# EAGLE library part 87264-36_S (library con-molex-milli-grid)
RECEPTACAL
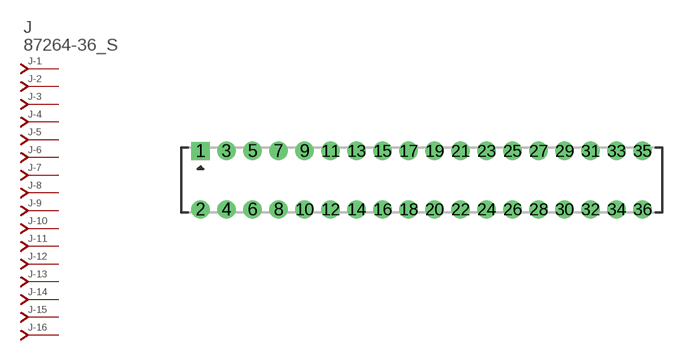
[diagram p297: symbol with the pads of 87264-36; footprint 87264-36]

Designator prefix J; gates -1=J-NV -2=J-N -3=J-N -4=J-N -5=J-N -6=J-N -7=J-N -8=J-N -9=J-N -10=J-N -11=J-N -12=J-N -13=J-N -14=J-N -15=J-N -16=J-N -17=J-N -18=J-N -19=J-N -20=J-N -21=J-N -22=J-N -23=J-N -24=J-N -25=J-N -26=J-N -27=J-N -28=J-N -29=J-N -30=J-N -31=J-N -32=J-N -33=J-N -34=J-N -35=J-N -36=J-N

## 87264-36_S  [87264-36]
1  -1:J  pas
2  -2:J  pas
3  -3:J  pas
4  -4:J  pas
5  -5:J  pas
6  -6:J  pas
7  -7:J  pas
8  -8:J  pas
9  -9:J  pas
10  -10:J  pas
11  -11:J  pas
12  -12:J  pas
13  -13:J  pas
14  -14:J  pas
15  -15:J  pas
16  -16:J  pas
17  -17:J  pas
18  -18:J  pas
19  -19:J  pas
20  -20:J  pas
21  -21:J  pas
22  -22:J  pas
23  -23:J  pas
24  -24:J  pas
25  -25:J  pas
26  -26:J  pas
27  -27:J  pas
28  -28:J  pas
29  -29:J  pas
30  -30:J  pas
31  -31:J  pas
32  -32:J  pas
33  -33:J  pas
34  -34:J  pas
35  -35:J  pas
36  -36:J  pas

## Footprint 87264-36 (pad centres in mm)
RECEPTACAL Dual Row, Side Entry
drill 0.914 square: 1 -17,2.25
drill 0.914: 2 -17,-2.25; 3 -15,2.25; 4 -15,-2.25; 5 -13,2.25; 6 -13,-2.25; 7 -11,2.25; 8 -11,-2.25; 9 -9,2.25; 10 -9,-2.25; 11 -7,2.25; 12 -7,-2.25; 13 -5,2.25; 14 -5,-2.25; 15 -3,2.25; 16 -3,-2.25; 17 -1,2.25; 18 -1,-2.25; 19 1,2.25; 20 1,-2.25; 21 3,2.25; 22 3,-2.25; 23 5,2.25; 24 5,-2.25; 25 7,2.25; 26 7,-2.25; 27 9,2.25; 28 9,-2.25; 29 11,2.25; 30 11,-2.25; 31 13,2.25; 32 13,-2.25; 33 15,2.25; 34 15,-2.25; 35 17,2.25; 36 17,-2.25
